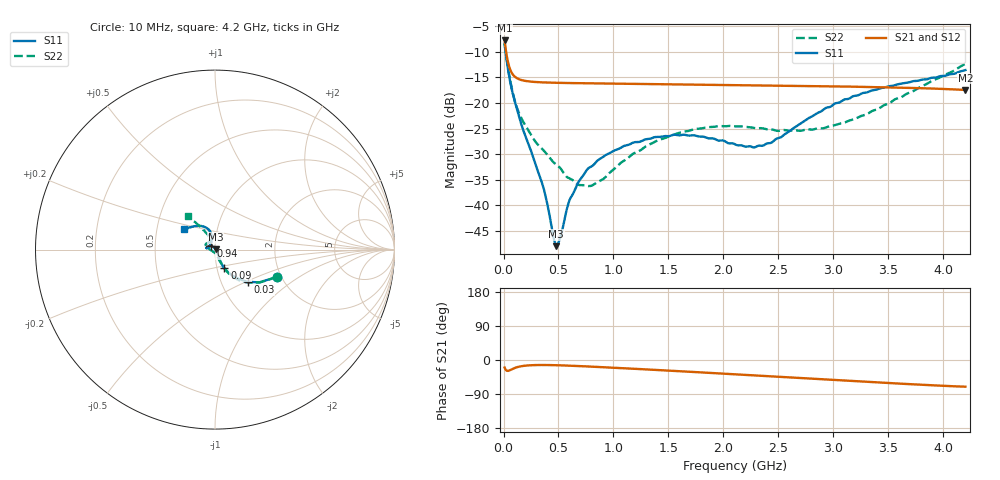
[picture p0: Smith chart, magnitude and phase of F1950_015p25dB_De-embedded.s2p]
! Integrated Device Technology
! Corporate Headquarters
! 6024 Silver Creek Valley Road
! San Jose, CA 95138  USA
! Phone:  1-408-284-8200
! Toll Free:  1-800-223-1366
! Webpage:  http://www.idt.com/
! Timing and RF Division
! 515 Groton Road, Suite 102
! Westford, MA 01886-6024
! Device:  F1950
! Description: 7-bit 0.25 dB Digital Step Attenuator
! Frequency:  150.0 -  4000.00 MHz
! Package:  4x4 mm Thin QFN Plastic Package: 24 pin
! Ports:  2 RF, 12 DC
!  Pin  1  = D0
!  Pin  2  = VDD
!  Pin  3  = Vmode
!  Pin  4  = GND
!  Pin  5  = RF1  =  Port 1
!  Pin  6  = GND
!  Pin  7  = GND
!  Pin  8  = GND
!  Pin  9  = GND
!  Pin 10  = GND
!  Pin 11  = GND
!  Pin 12  = GND
!  Pin 13  = GND
!  Pin 14  = RF2  =  Port 2
!  Pin 15  = GND
!  Pin 16  = LE
!  Pin 17  = CLK
!  Pin 18  = DATE
!  Pin 19  = D6
!  Pin 20  = D5
!  Pin 21  = D4
!  Pin 22  = D3
!  Pin 23  = D2
!  Pin 24  = D1
! State:  61
! Atten State:  15.25 dB
! Voltage:  +5.00 Volts
! Current:  Not Measured mA
! Data:  The device was measured on a the F195X evaluation board which has
!  individual transmission lines to the RF pins.  Data was collected
!  using a calibrated network analyzer.  The evaluation board was
!  de-embedded using a TRL calibration technique.
!  The reference plane is the edge of the package pin.
! Misc:  Board 2019
!  Action Tracker AT0250
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# GHz S dB R 50
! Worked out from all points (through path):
!   420 points, 10 MHz to 4.2 GHz, reference 50 ohm
!   highest |S21| = -7.81 dB at 10 MHz (marker M1); lowest = -17.5 dB at 4.2 GHz (marker M2)
!   group delay of S21, straight-line fit = 40.8 ps
!   lowest |S11| = -47.9 dB at 480 MHz (marker M3), VSWR 1.01, Z = 50.3 + j0.225 ohm
!   |S11| at or under -10 dB: 18.72 MHz to end of sweep
!   |S22| runs from -36.2 to -8.5 dB; largest |S21 - S12| = 0.00023
!   S11 on the Smith chart (normalised r, x): 10 MHz: 1.90, -0.67; 30 MHz: 1.34, -0.51; 90 MHz: 1.08, -0.23; 940 MHz: 0.95, +0.04; 4.2 GHz: 0.69, +0.16
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0.01  -8.44 -23.6  -7.81 -19.8  -7.81 -19.8  -8.48 -24.1
0.03  -11.82 -44.4  -10.88 -28.4  -10.87 -28.4  -11.73 -45.1
0.05  -14.61 -54.5  -12.80 -27.9  -12.80 -27.9  -14.37 -55.5
0.09  -18.69 -63.4  -14.59 -22.5  -14.59 -22.4  -18.53 -62.8
0.15  -23.32 -65.0  -15.44 -17.1  -15.44 -17.1  -22.43 -67.0
0.26  -29.96 -58.1  -15.87 -13.7  -15.86 -13.7  -26.56 -69.3
0.36  -36.34 -45.2  -15.99 -13.2  -15.99 -13.2  -29.16 -72.8
0.46  -46.73 3.6  -16.06 -13.6  -16.06 -13.6  -31.69 -78.4
0.48  -47.94 33.9  -16.07 -13.8  -16.07 -13.8  -32.04 -80.7
0.52  -45.87 82.0  -16.09 -14.1  -16.09 -14.1  -32.82 -82.7
0.6  -38.96 113.8  -16.12 -14.9  -16.12 -15.0  -34.73 -95.1
0.71  -34.60 126.2  -16.15 -16.3  -16.15 -16.3  -36.04 -115.2
0.8  -32.39 132.7  -16.18 -17.5  -16.18 -17.5  -36.15 -136.0
0.94  -30.05 141.5  -16.23 -19.5  -16.22 -19.5  -34.20 -162.6
1.41  -26.63 163.9  -16.35 -26.6  -16.34 -26.6  -27.25 166.1
1.73  -26.31 170.9  -16.42 -31.6  -16.42 -31.6  -25.14 157.2
2.11  -28.12 160.5  -16.51 -37.9  -16.51 -37.9  -24.58 147.5
2.43  -27.81 125.3  -16.59 -43.0  -16.59 -43.1  -25.17 137.1
2.81  -22.58 103.7  -16.70 -49.4  -16.69 -49.5  -25.19 121.4
3.1  -19.32 106.1  -16.79 -54.3  -16.79 -54.4  -23.82 116.1
3.51  -16.72 117.3  -16.97 -60.9  -16.96 -60.9  -20.04 117.2
4.2  -13.59 146.8  -17.46 -70.4  -17.46 -70.5  -12.38 129.2
